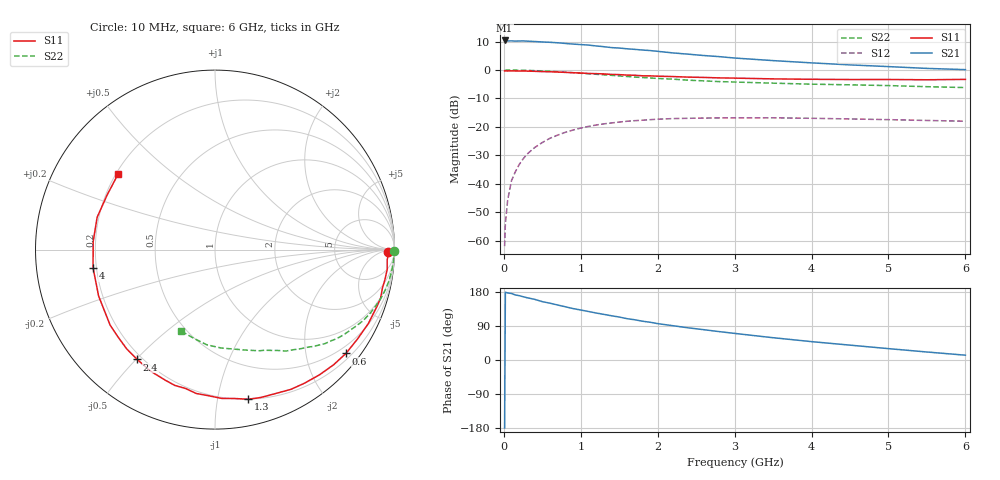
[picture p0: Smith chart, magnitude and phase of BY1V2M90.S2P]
! SIEMENS Small Signal Semiconductors
! BFY420
! Si NPN RF SIEGET Grounded Emitter Transistor in MICRO-X
! VCE = 1.25 V  IC = 0.9 mA
! Common Emitter S-Parameters:  October  1996
# GHz  S  MA  R  50
!  f  S11  S21  S12  S22
! GHz  MAG  ANG  MAG  ANG  MAG  ANG  MAG  ANG
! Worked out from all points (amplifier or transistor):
!   36 points, 10 MHz to 6 GHz, reference 50 ohm
!   highest |S21| = 10.4 dB at 10 MHz (marker M1)
!   |S21| within 3 dB of that: start of sweep to 1.636 GHz
!   unconditionally stable (mu >= 1): 4.588 GHz to end of sweep
!   at 250 MHz: K = 0.03, MSG = 20.8 dB, |S12| = -31.3 dB
!   at 1.4 GHz: K = 0.22, MSG = 13.2 dB, |S12| = -18.6 dB
!   at 6 GHz: K = 1.34, MAG = 5.6 dB, |S12| = -18.0 dB
!   S11 on the Smith chart (normalised r, x): 10 MHz: 46, -17; 600 MHz: 0.33, -2.84; 1.3 GHz: 0.20, -1.23; 2.4 GHz: 0.18, -0.50; 4 GHz: 0.19, -0.07; 6 GHz: 0.21, +0.33
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0.01  0.9624 -0.8  3.307 -179.4  0.0008 107.4  0.9999 -0.4
0.02  0.9672 -1.5  3.303 178.6  0.002 83.9  0.99 -0.6
0.05  0.961 -3.3  3.241 177.0  0.0052 89.4  0.9967 -1.7
0.1  0.9658 -6.6  3.255 175.4  0.0114 86.5  0.9964 -3.4
0.15  0.9615 -9.9  3.221 171.6  0.0163 83.5  0.9942 -5.1
0.3  0.9564 -19.3  3.217 164.4  0.033 78.2  0.9854 -10.1
0.4  0.9487 -25.7  3.169 160.1  0.0433 74.3  0.9749 -13.4
0.5  0.9374 -32.0  3.113 154.0  0.0531 69.8  0.9625 -16.6
0.6  0.9312 -38.4  3.069 149.9  0.0631 66.3  0.9477 -19.7
0.9  0.8962 -56.1  2.857 135.7  0.088 55.1  0.8957 -28.2
1.1  0.8696 -67.4  2.744 128.0  0.102 48.4  0.8589 -33.6
1.3  0.854 -77.5  2.569 120.4  0.1131 42.1  0.8222 -38.2
1.6  0.8141 -92.9  2.361 109.1  0.1256 34.2  0.7695 -44.5
1.8  0.7912 -101.9  2.246 102.4  0.131 29.3  0.7381 -48.0
2.2  0.7664 -118.0  1.995 90.4  0.14 20.8  0.69 -55.0
2.4  0.75 -125.3  1.897 84.8  0.1416 17.4  0.662 -58.1
2.8  0.7269 -138.2  1.717 74.9  0.1439 11.1  0.6255 -63.7
3.5  0.6981 -158.3  1.463 58.8  0.1445 2.9  0.5869 -72.6
4  0.6869 -171.5  1.335 48.5  0.1416 -1.8  0.5636 -79.5
4.5  0.6802 176.3  1.23 39.2  0.138 -5.7  0.5488 -86.6
5.5  0.6736 153.1  1.067 21.1  0.1297 -9.9  0.5089 -103.2
6  0.6842 142.2  1.015 12.7  0.1258 -9.9  0.4914 -112.6
